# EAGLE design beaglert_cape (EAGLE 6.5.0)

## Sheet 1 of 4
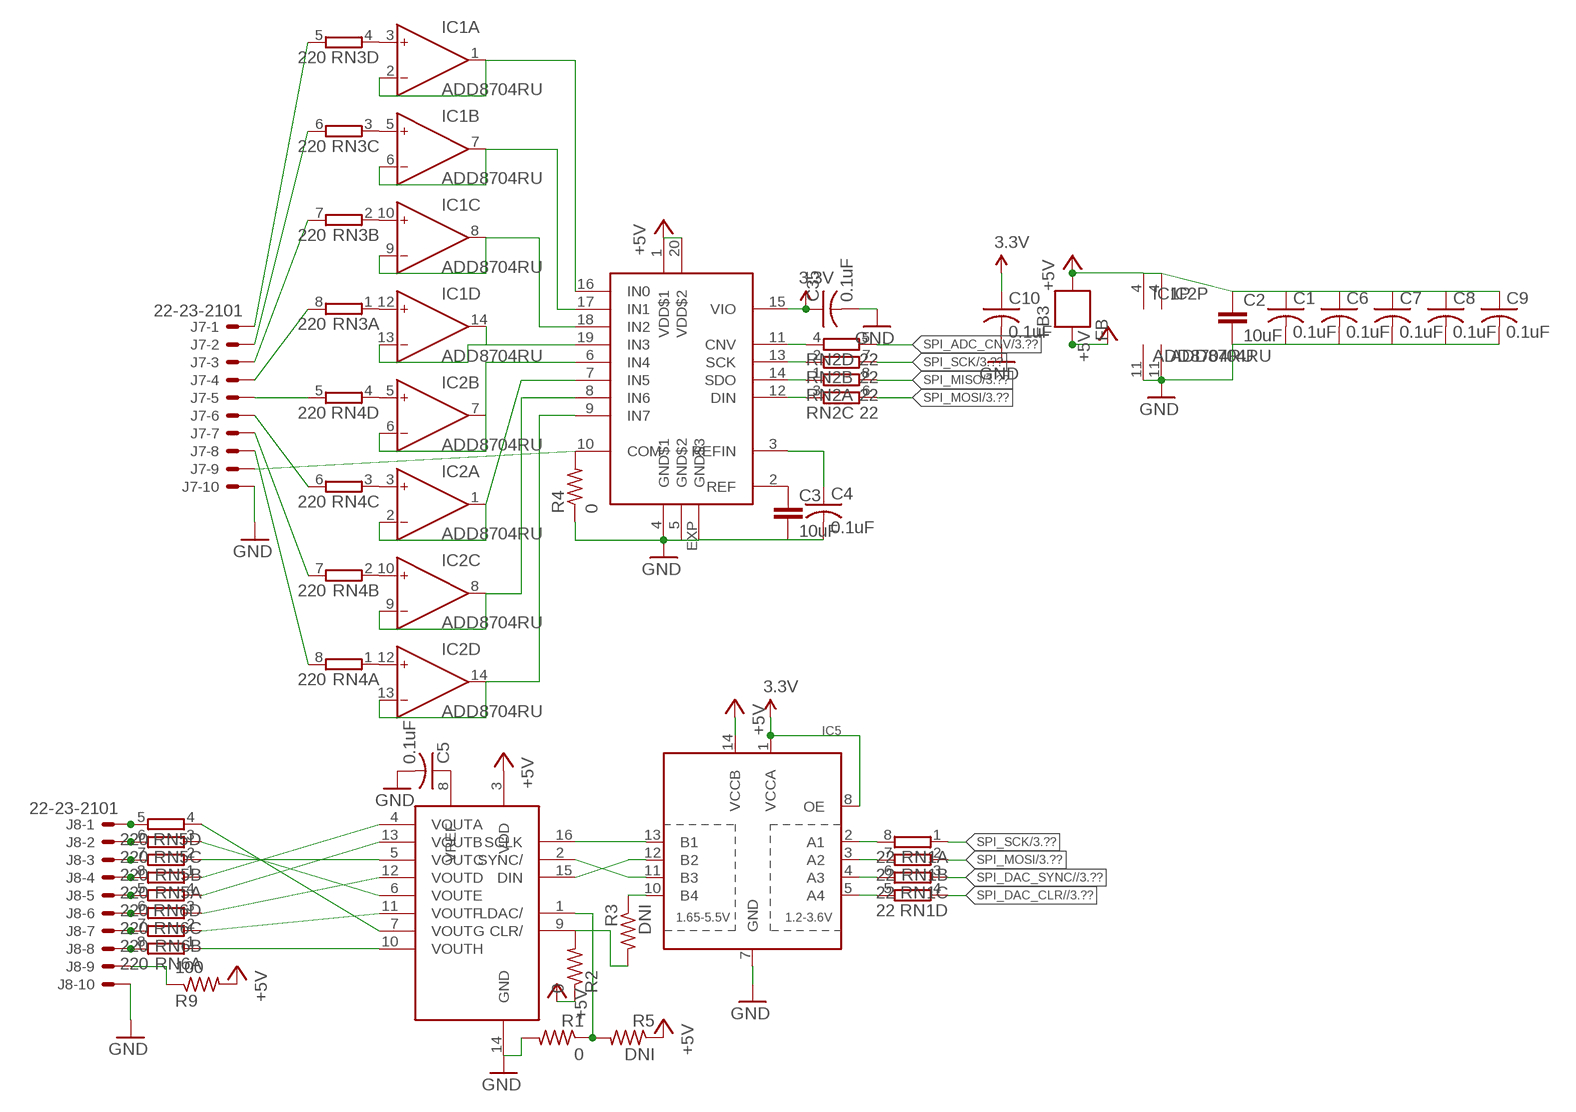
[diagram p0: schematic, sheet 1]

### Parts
C1  0.1uF  C-USC0603  [C0603]
C2  10uF  CAP0603-CAP  [0603-CAP]
C3  10uF  CAP0603-CAP  [0603-CAP]
C4  0.1uF  C-USC0603  [C0603]
C5  0.1uF  C-USC0603  [C0603]
C6  0.1uF  C-USC0603  [C0603]
C7  0.1uF  C-USC0603  [C0603]
C8  0.1uF  C-USC0603  [C0603]
C9  0.1uF  C-USC0603  [C0603]
C10  0.1uF  C-USC0603  [C0603]
C35  0.1uF  C-USC0603  [C0603]
FB3  FB  [0603]
IC1  ADD8704RU  [TSSOP14]
IC2  ADD8704RU  [TSSOP14]
IC3  AD5668  [TSSOP16-PW]
IC4  AD7699  [LFCSP20-LEADS]
IC5  TXB0104PWR  [TSSOP14]
J7  22-23-2101  [22-23-2101]
J8  22-23-2101  [22-23-2101]
R1  0  R-US_R0603  [R0603]
R2  0  R-US_R0603  [R0603]
R3  DNI  R-US_R0603  [R0603]
R4  0  R-US_R0603  [R0603]
R5  DNI  R-US_R0603  [R0603]
R9  100  R-US_R0603  [R0603]
RN1  22  4R-N0603-ARC  [0603-ARC]
RN2  22  4R-N0603-ARC  [0603-ARC]
RN3  220  4R-N0603-ARC  [0603-ARC]
RN4  220  4R-N0603-ARC  [0603-ARC]
RN5  220  4R-N0603-ARC  [0603-ARC]
RN6  220  4R-N0603-ARC  [0603-ARC]

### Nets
3.3V: C10.1 C35.1 IC4.15(VIO) IC5.1(VCCA) IC5.8(OE) ; also sheet 3,4
+5V_ADC_DAC: C1.1 C2.1 C6.1 C7.1 C8.1 C9.1 FB3.1 IC1.4(P:V+) IC2.4(P:V+) IC3.3(VDD) IC4.1(VDD$1) IC4.20(VDD$2) IC5.14(VCCB) R2.1 R5.1 R9.2 ; supply symbol labelled +5V
+5V_SYS: FB3.2 ; supply symbol labelled +5V ; also sheet 3
DGND: C1.2 C2.2 C3.2 C4.2 C5.2 C6.2 C7.2 C8.2 C9.2 C10.2 C35.2 IC1.11(P:V-) IC2.11(P:V-) IC3.14(GND) IC4.4(GND$1) IC4.5(GND$2) IC4.EXP(GND$3) IC5.7(GND) J7.10 J8.10 R1.2 R4.1 ; supply symbol labelled GND ; also sheet 3,4
N$1: IC3.16(SCLK) IC5.13(B1)
N$2: IC3.15(DIN) IC5.12(B2)
N$3: IC3.2(SYNC/) IC5.11(B3)
N$4: IC3.9(CLR/) R2.2 R3.2
N$5: IC1.1(A:OUT) IC1.2(A:IN-) IC4.16(IN0)
N$6: IC1.6(B:IN-) IC1.7(B:OUT) IC4.17(IN1)
N$7: IC1.8(C:OUT) IC1.9(C:IN-) IC4.18(IN2)
N$8: IC1.13(D:IN-) IC1.14(D:OUT) IC4.19(IN3)
N$9: IC2.1(A:OUT) IC2.2(A:IN-) IC4.7(IN5)
N$10: IC2.6(B:IN-) IC2.7(B:OUT) IC4.6(IN4)
N$11: IC2.8(C:OUT) IC2.9(C:IN-) IC4.8(IN6)
N$12: IC2.13(D:IN-) IC2.14(D:OUT) IC4.9(IN7)
N$13: IC5.10(B4) R3.1
N$14: IC4.11(CNV) RN2.4
N$15: C5.1 IC3.8(VREF)
N$16: IC5.2(A1) RN1.8
N$17: IC5.3(A2) RN1.7
N$18: IC5.4(A3) RN1.6
N$19: IC5.5(A4) RN1.5
N$20: IC4.12(DIN) RN2.3
N$21: C3.1 IC4.2(REF)
N$22: C4.1 IC4.3(REFIN)
N$23: IC4.13(SCK) RN2.2
N$24: IC4.14(SDO) RN2.1
N$25: IC4.10(COM) J7.9 R4.2
N$27: IC1.3(A:IN+) RN3.4
N$29: IC1.5(B:IN+) RN3.3
N$30: IC1.10(C:IN+) RN3.2
N$31: IC1.12(D:IN+) RN3.1
N$32: IC2.5(B:IN+) RN4.4
N$33: IC2.3(A:IN+) RN4.3
N$34: IC2.10(C:IN+) RN4.2
N$35: IC2.12(D:IN+) RN4.1
N$36: IC3.1(LDAC/) R1.1 R5.2
N$37: J7.1 RN3.5
N$38: J7.2 RN3.6
N$39: J7.3 RN3.7
N$40: J7.4 RN3.8
N$41: J7.5 RN4.5
N$42: J7.6 RN4.6
N$43: J7.7 RN4.7
N$44: J7.8 RN4.8
N$45: IC3.7(VOUTG) RN5.4
N$46: IC3.6(VOUTE) RN5.3
N$47: IC3.5(VOUTC) RN5.2
N$48: IC3.4(VOUTA) RN5.1
N$49: IC3.13(VOUTB) RN6.4
N$50: IC3.12(VOUTD) RN6.3
N$51: IC3.11(VOUTF) RN6.2
N$52: J8.8 RN6.8
N$61: J8.9 R9.1
N$72: IC3.10(VOUTH) RN6.1
N$73: J8.7 RN6.7
N$74: J8.6 RN6.6
N$75: J8.5 RN6.5
N$76: J8.4 RN5.8
N$77: J8.3 RN5.7
N$78: J8.2 RN5.6
N$79: J8.1 RN5.5
SPI_ADC_CNV: RN2.5 ; also sheet 3
SPI_DAC_CLR/: RN1.4 ; also sheet 3
SPI_DAC_SYNC/: RN1.3 ; also sheet 3
SPI_MISO: RN2.8 ; also sheet 3
SPI_MOSI: RN1.2 RN2.6 ; also sheet 3
SPI_SCK: RN1.1 RN2.7 ; also sheet 3

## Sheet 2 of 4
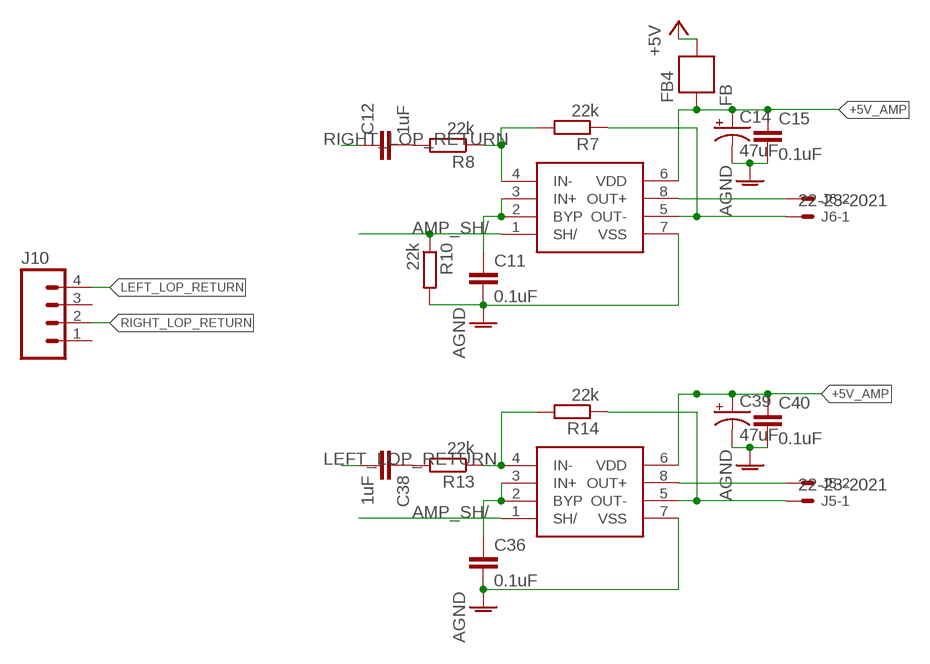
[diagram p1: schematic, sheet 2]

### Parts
C11  0.1uF  C-EUC0603  [C0603]
C12  1uF  C-EUC0603  [C0603]
C14  47uF  CAP_POL1206  [EIA3216]
C15  0.1uF  C-EUC0603  [C0603]
C36  0.1uF  C-EUC0603  [C0603]
C38  1uF  C-EUC0603  [C0603]
C39  47uF  CAP_POL1206  [EIA3216]
C40  0.1uF  C-EUC0603  [C0603]
FB4  FB  [0603]
IC8  LM4876  [SO8]
IC9  LM4876  [SO8]
J5  22-23-2021  [22-23-2021]
J6  22-23-2021  [22-23-2021]
J10  M04PTH  [1X04]
R7  22k  R-EU_R0603  [R0603]
R8  22k  R-EU_R0603  [R0603]
R10  22k  R-EU_R0603  [R0603]
R13  22k  R-EU_R0603  [R0603]
R14  22k  R-EU_R0603  [R0603]

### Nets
+5V_AMP: C14.A(+) C15.1 C39.A(+) C40.1 FB4.2 IC8.6(VDD) IC9.6(VDD)
+5V_POW: FB4.1 ; supply symbol labelled +5V ; also sheet 3
AGND: C11.2 C14.C(-) C15.2 C36.2 C39.C(-) C40.2 IC8.7(VSS) IC9.7(VSS) R10.2 ; also sheet 3
AMP_SH/: IC8.1(SH/) IC9.1(SH/) R10.1 ; also sheet 3
LEFT_LOP_RETURN: C38.2 J10.4
N$26: IC9.4(IN-) R13.1 R14.2
N$28: IC8.4(IN-) R7.2 R8.1
N$53: C11.1 IC8.2(BYP) IC8.3(IN+)
N$55: C12.2 R8.2
N$57: IC8.5(OUT-) J6.1 R7.1
N$60: C36.1 IC9.2(BYP) IC9.3(IN+)
N$64: C38.1 R13.2
N$65: IC9.5(OUT-) J5.1 R14.1
N$67: IC9.8(OUT+) J5.2
N$71: IC8.8(OUT+) J6.2
RIGHT_LOP_RETURN: C12.1 J10.2
Unconnected: J10.1 J10.3

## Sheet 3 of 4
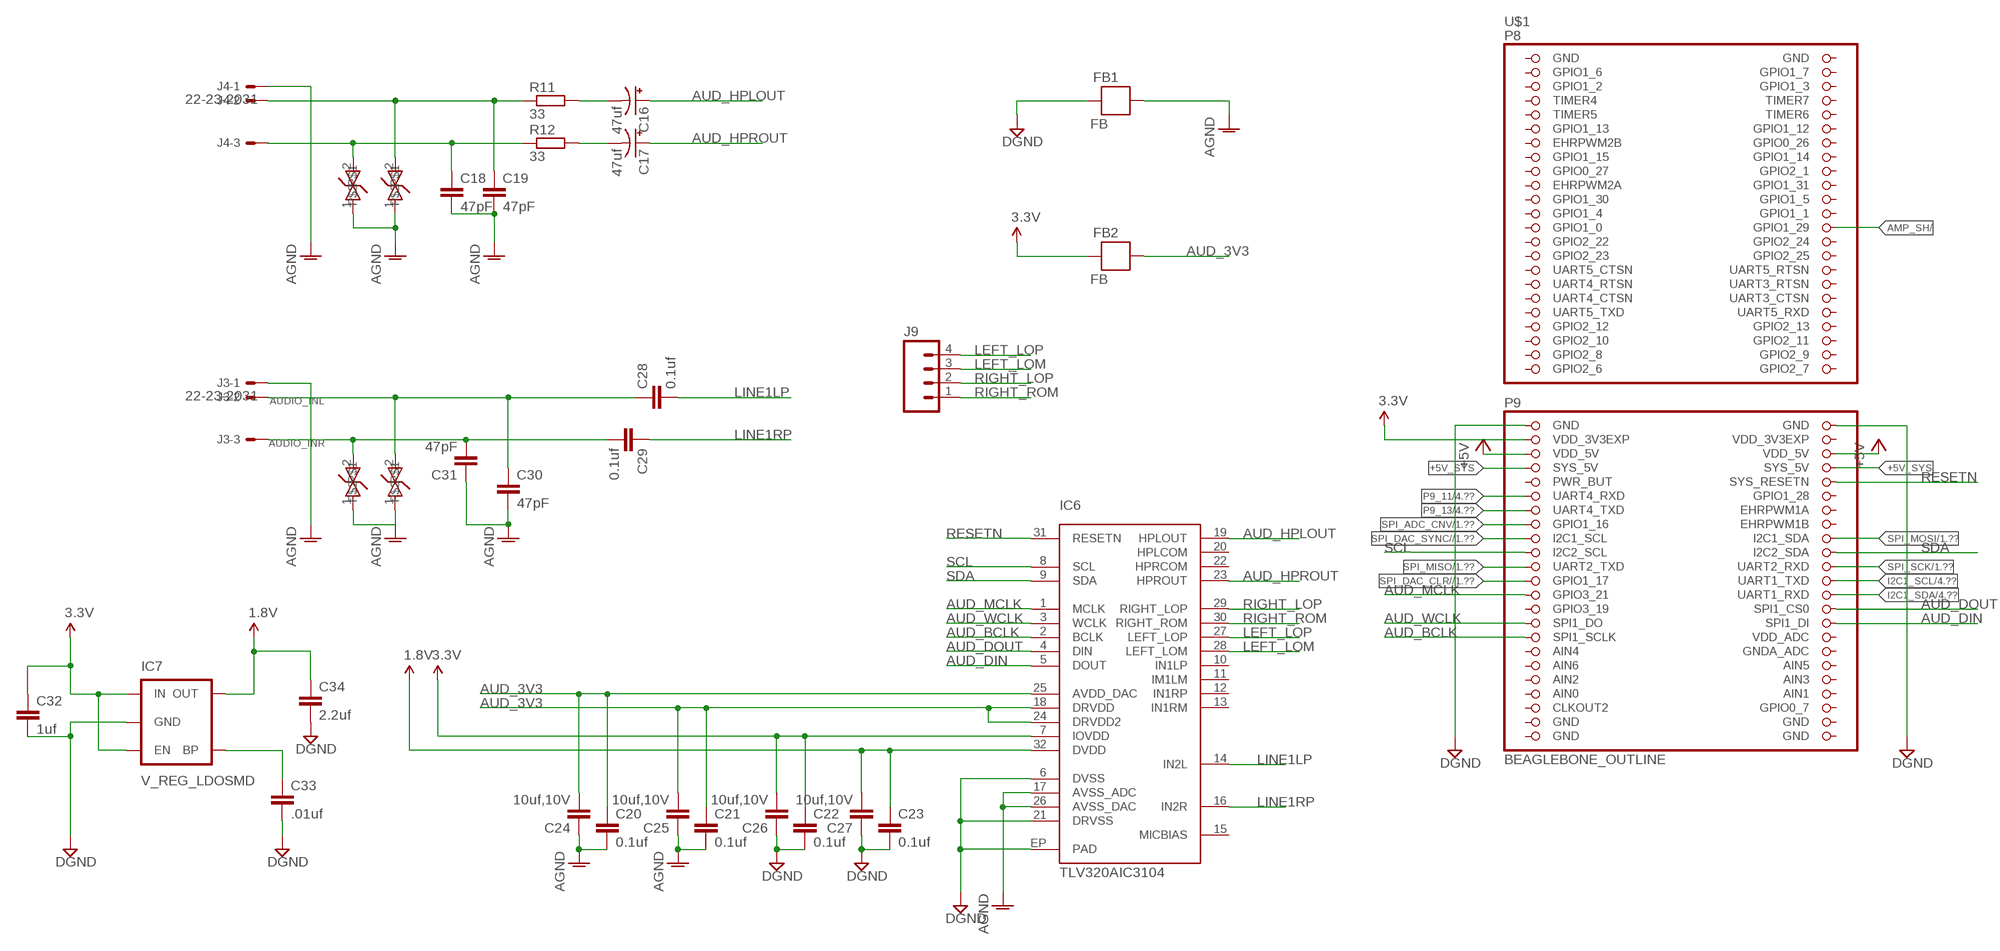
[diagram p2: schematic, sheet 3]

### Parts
C16  47uf  CAP_POL1206  [EIA3216]
C17  47uf  CAP_POL1206  [EIA3216]
C18  47pF  C-EUC0603  [C0603]
C19  47pF  C-EUC0603  [C0603]
C20  0.1uf  C-EUC0603  [C0603]
C21  0.1uf  C-EUC0603  [C0603]
C22  0.1uf  C-EUC0603  [C0603]
C23  0.1uf  C-EUC0603  [C0603]
C24  10uf,10V  CAP0603-CAP  [0603-CAP]
C25  10uf,10V  CAP0603-CAP  [0603-CAP]
C26  10uf,10V  CAP0603-CAP  [0603-CAP]
C27  10uf,10V  CAP0603-CAP  [0603-CAP]
C28  0.1uf  C-EUC0603  [C0603]
C29  0.1uf  C-EUC0603  [C0603]
C30  47pF  C-EUC0603  [C0603]
C31  47pF  C-EUC0603  [C0603]
C32  1uf  C-EUC0603  [C0603]
C33  .01uf  C-EUC0603  [C0603]
C34  2.2uf  C-EUC0603  [C0603]
D1  PGB0010603MR  [0603]
D2  PGB0010603MR  [0603]
D3  PGB0010603MR  [0603]
D4  PGB0010603MR  [0603]
FB1  FB  [0603]
FB2  FB  [0603]
IC6  TLV320AIC3104  [QFN-32]
IC7  V_REG_LDOSMD  [SOT23-5]
J3  22-23-2031  [22-23-2031]
J4  22-23-2031  [22-23-2031]
J9  M04PTH  [1X04]
R11  33  R-EU_R0603  [R0603]
R12  33  R-EU_R0603  [R0603]
U$1  BEAGLEBONE_OUTLINE  [BEAGLEBONE_SHIELD]

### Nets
1.8V: C23.1 C27.2 C34.1 IC6.32(DVDD) IC7.5(OUT)
3.3V: C22.1 C26.2 C32.1 FB2.2 IC6.7(IOVDD) IC7.1(IN) IC7.3(EN) U$1.49(VDD_3V3EXP) ; also sheet 1,4
+5V_POW: U$1.51(VDD_5V) U$1.52(VDD_5V) ; supply symbol labelled +5V ; also sheet 2
+5V_SYS: U$1.53(SYS_5V) U$1.54(SYS_5V) ; also sheet 1
AGND: C18.2 C19.2 C20.2 C21.2 C24.1 C25.1 C30.2 C31.1 D1.1 D2.1 D3.1 D4.1 FB1.1 IC6.17(AVSS_ADC) IC6.26(AVSS_DAC) J3.1 J4.1 ; also sheet 2
AMP_SH/: U$1.26(GPIO1_29) ; also sheet 2
AUD_3V3: C20.1 C21.1 C24.2 C25.2 FB2.1 IC6.18(DRVDD) IC6.24(DRVDD2) IC6.25(AVDD_DAC)
AUD_BCLK: IC6.2(BCLK) U$1.77(SPI1_SCLK)
AUD_DIN: IC6.5(DOUT) U$1.76(SPI1_DI)
AUD_DOUT: IC6.4(DIN) U$1.74(SPI1_CS0)
AUD_HPLOUT: C16.A(+) IC6.19(HPLOUT)
AUD_HPROUT: C17.A(+) IC6.23(HPROUT)
AUD_MCLK: IC6.1(MCLK) U$1.71(GPIO3_21)
AUD_WCLK: IC6.3(WCLK) U$1.75(SPI1_DO)
AUDIO_INL: C28.1 C30.1 D4.2 J3.2
AUDIO_INR: C29.2 C31.2 D3.2 J3.3
DGND: C22.2 C23.2 C26.1 C27.1 C32.2 C33.2 C34.2 FB1.2 IC6.6(DVSS) IC6.21(DRVSS) IC6.EP(PAD) IC7.2(GND) U$1.47(GND) U$1.48(GND) ; also sheet 1,4
HPL: C19.1 D2.2 J4.2 R11.1
HPR: C18.1 D1.2 J4.3 R12.1
I2C1_SCL: U$1.70(UART1_TXD) ; also sheet 4
I2C1_SDA: U$1.72(UART1_RXD) ; also sheet 4
LEFT_LOM: IC6.28(LEFT_LOM) J9.3
LEFT_LOP: IC6.27(LEFT_LOP) J9.4
LINE1LP: C28.2 IC6.14(IN2L)
LINE1RP: C29.1 IC6.16(IN2R)
N$54: C16.C(-) R11.2
N$59: C17.C(-) R12.2
N$63: C33.1 IC7.4(BP)
P9_11: U$1.57(UART4_RXD) ; also sheet 4
P9_13: U$1.59(UART4_TXD) ; also sheet 4
RESETN: IC6.31(RESETN) U$1.56(SYS_RESETN)
RIGHT_LOP: IC6.29(RIGHT_LOP) J9.2
RIGHT_ROM: IC6.30(RIGHT_ROM) J9.1
SCL: IC6.8(SCL) U$1.65(I2C2_SCL)
SDA: IC6.9(SDA) U$1.66(I2C2_SDA)
SPI_ADC_CNV: U$1.61(GPIO1_16) ; also sheet 1
SPI_DAC_CLR/: U$1.69(GPIO1_17) ; also sheet 1
SPI_DAC_SYNC/: U$1.63(I2C1_SCL) ; also sheet 1
SPI_MISO: U$1.67(UART2_TXD) ; also sheet 1
SPI_MOSI: U$1.64(I2C1_SDA) ; also sheet 1
SPI_SCK: U$1.68(UART2_RXD) ; also sheet 1
Unconnected: IC6.10(IN1LP) IC6.11(IM1LM) IC6.12(IN1RP) IC6.13(IN1RM) IC6.15(MICBIAS) IC6.20(HPLCOM) IC6.22(HPRCOM) U$1.3(GPIO1_6) U$1.4(GPIO1_7) U$1.5(GPIO1_2) U$1.6(GPIO1_3) U$1.7(TIMER4) U$1.8(TIMER7) U$1.9(TIMER5) U$1.10(TIMER6) U$1.11(GPIO1_13) U$1.12(GPIO1_12) U$1.13(EHRPWM2B) U$1.14(GPIO0_26) U$1.15(GPIO1_15) U$1.16(GPIO1_14) U$1.17(GPIO0_27) U$1.18(GPIO2_1) U$1.19(EHRPWM2A) U$1.20(GPIO1_31) U$1.21(GPIO1_30) U$1.22(GPIO1_5) U$1.23(GPIO1_4) U$1.24(GPIO1_1) U$1.25(GPIO1_0) U$1.27(GPIO2_22) U$1.28(GPIO2_24) U$1.29(GPIO2_23) U$1.30(GPIO2_25) U$1.31(UART5_CTSN) U$1.32(UART5_RTSN) U$1.33(UART4_RTSN) U$1.34(UART3_RTSN) U$1.35(UART4_CTSN) U$1.36(UART3_CTSN) U$1.37(UART5_TXD) U$1.38(UART5_RXD) U$1.39(GPIO2_12) U$1.40(GPIO2_13) U$1.41(GPIO2_10) U$1.42(GPIO2_11) U$1.43(GPIO2_8) U$1.44(GPIO2_9) U$1.45(GPIO2_6) U$1.46(GPIO2_7) U$1.55(PWR_BUT) U$1.58(GPIO1_28) U$1.60(EHRPWM1A) U$1.62(EHRPWM1B) U$1.73(GPIO3_19) U$1.78(VDD_ADC) U$1.79(AIN4) U$1.80(GNDA_ADC) U$1.81(AIN6) U$1.82(AIN5) U$1.83(AIN2) U$1.84(AIN3) U$1.86(AIN1) U$1.87(CLKOUT2) U$1.88(GPIO0_7)

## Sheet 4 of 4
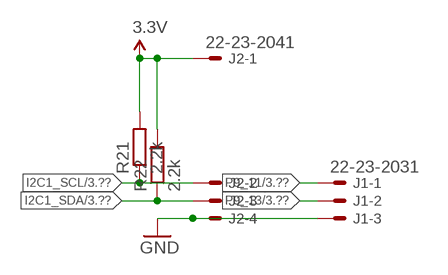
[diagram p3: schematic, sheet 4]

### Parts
J1  22-23-2031  [22-23-2031]
J2  22-23-2041  [22-23-2041]
R21  2.2k  R-EU_R0603  [R0603]
R22  2.2k  R-EU_R0603  [R0603]

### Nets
3.3V: J2.1 R21.2 R22.2 ; also sheet 1,3
DGND: J1.3 J2.4 ; supply symbol labelled GND ; also sheet 1,3
I2C1_SCL: J2.2 R21.1 ; also sheet 3
I2C1_SDA: J2.3 R22.1 ; also sheet 3
P9_11: J1.1 ; also sheet 3
P9_13: J1.2 ; also sheet 3

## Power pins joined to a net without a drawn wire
AIN0: U$1.85(AIN0)
DGND: U$1.1(GND) U$1.2(GND) U$1.89(GND) U$1.90(GND) U$1.91(GND) U$1.92(GND)
VDD_3V3EXP: U$1.50(VDD_3V3EXP)

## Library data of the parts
C1 C4-C10 C35 = rcl:C-US: CAPACITOR, American symbol
C2 C3 = SparkFun-Passives:CAP: Capacitor
C11 C12 C15 C36 C38 C40 = rcl:C-EU: CAPACITOR, European symbol
C14 C39 = SparkFun-Capacitors:CAP_POL: Capacitor Polarized
C16 C17 = SparkFun-Capacitors:CAP_POL: Capacitor Polarized; MANEX: 123-0001196
C18 C19 C30 C31 = rcl:C-EU: CAPACITOR, European symbol; MANEX: 123-0001115
C20-C23 = rcl:C-EU: CAPACITOR, European symbol; MANEX: 123-0001056
C24-C27 = SparkFun-Passives:CAP: Capacitor; MANEX: 123-0001127
C28 C29 C33 = rcl:C-EU: CAPACITOR, European symbol; MANEX: 123-0001032
C32 = rcl:C-EU: CAPACITOR, European symbol; MANEX: 123-0001087
C34 = rcl:C-EU: CAPACITOR, European symbol; MANEX: 123-0001094
D1-D4 = CircuitCo:PGB0010603MR; MANEX: 130-0001371
FB1 FB2 = SparkFun-Passives:FB; MANEX: 126-0001418
FB3 FB4 = SparkFun-Passives:FB
IC1 IC2 = analog-devices:ADD8704: 16 V Quad Operational Amplifier Source: Ananlog Devices .. 780914713ADD8704_0.pdf; MF: ALTERA CORPORATION; MPN: ADD8704ARUZ-REEL; OC_FARNELL: unknown; OC_NEWARK: 59K0964
IC3 = custom:AD5668
IC4 = custom:AD7699
IC5 = SparkFun-DigitalIC:TXB0104PWR: 4-Bit Bi-Directional Level Shifter 1.2V-3.6V (VCCA) to 1.65V-5.5V (VCCB) bi-directional level shifter with auto direction sensing. Max data rate - VCCA 1.8V: 20Mbps (50ns), VCCA 3.3V: 100Mbps (10ns) Digikey: 296-21929-1-ND (TSSOP) IC-11329
IC6 = CircuitCo:TLV320AIC3104; MANEX: 140-0004277
IC7 = SparkFun-PowerIC:V_REG_LDO: Voltage Regulator LDO Standard 150mA LDO voltage regulator in SOT-23 layout. Micrel part MIC5205. BP (by-pass) pin is used to lower output noise with 470pF cap.; MANEX: 140-0001616
IC8 IC9 = custom:LM4876
J1 J3 J4 = con-molex:22-23-2031: .100" (2.54mm) Center Header - 3 Pin; MF: MOLEX; MPN: 22-23-2031; OC_FARNELL: 1462950; OC_NEWARK: 30C0862
J2 = con-molex:22-23-2041: .100" (2.54mm) Center Header - 4 Pin; MF: MOLEX; MPN: 22-23-2041; OC_FARNELL: 1462920; OC_NEWARK: 38C0355
J5 J6 = con-molex:22-23-2021: .100" (2.54mm) Center Header - 2 Pin; MF: MOLEX; MPN: 22-23-2021; OC_FARNELL: 1462926; OC_NEWARK: 25C3832
J7 J8 = con-molex:22-23-2101: .100" (2.54mm) Center Header - 10 Pin; MF: MOLEX; MPN: 22-23-2101; OC_FARNELL: 1756828; OC_NEWARK: 94C0765
J9 J10 = SparkFun-Connectors:M04: Header 4 Standard 4-pin 0.1" header. Use with straight break away headers (SKU : PRT-00116), right angle break away headers (PRT-00553), swiss pins (PRT-00743), machine pins (PRT-00117), and female headers (PRT-00115). Molex polarized connector foot print use with SKU : PRT-08231 with associated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; MANEX: 258-0002845
R1-R5 R9 = rcl:R-US_: RESISTOR, American symbol
R7 R8 R10 R13 R14 R21 R22 = rcl:R-EU_: RESISTOR, European symbol
R11 R12 = rcl:R-EU_: RESISTOR, European symbol; MANEX: 110-0002014
RN1-RN6 = resistor-dil:4R-N: Array Chip Resistor Source: RS Component / Phycomp; OC_FARNELL: unknown; OC_NEWARK: unknown
U$1 = adafruit:BEAGLEBONE_OUTLINE: Should match A3 pinout - but not completely tested

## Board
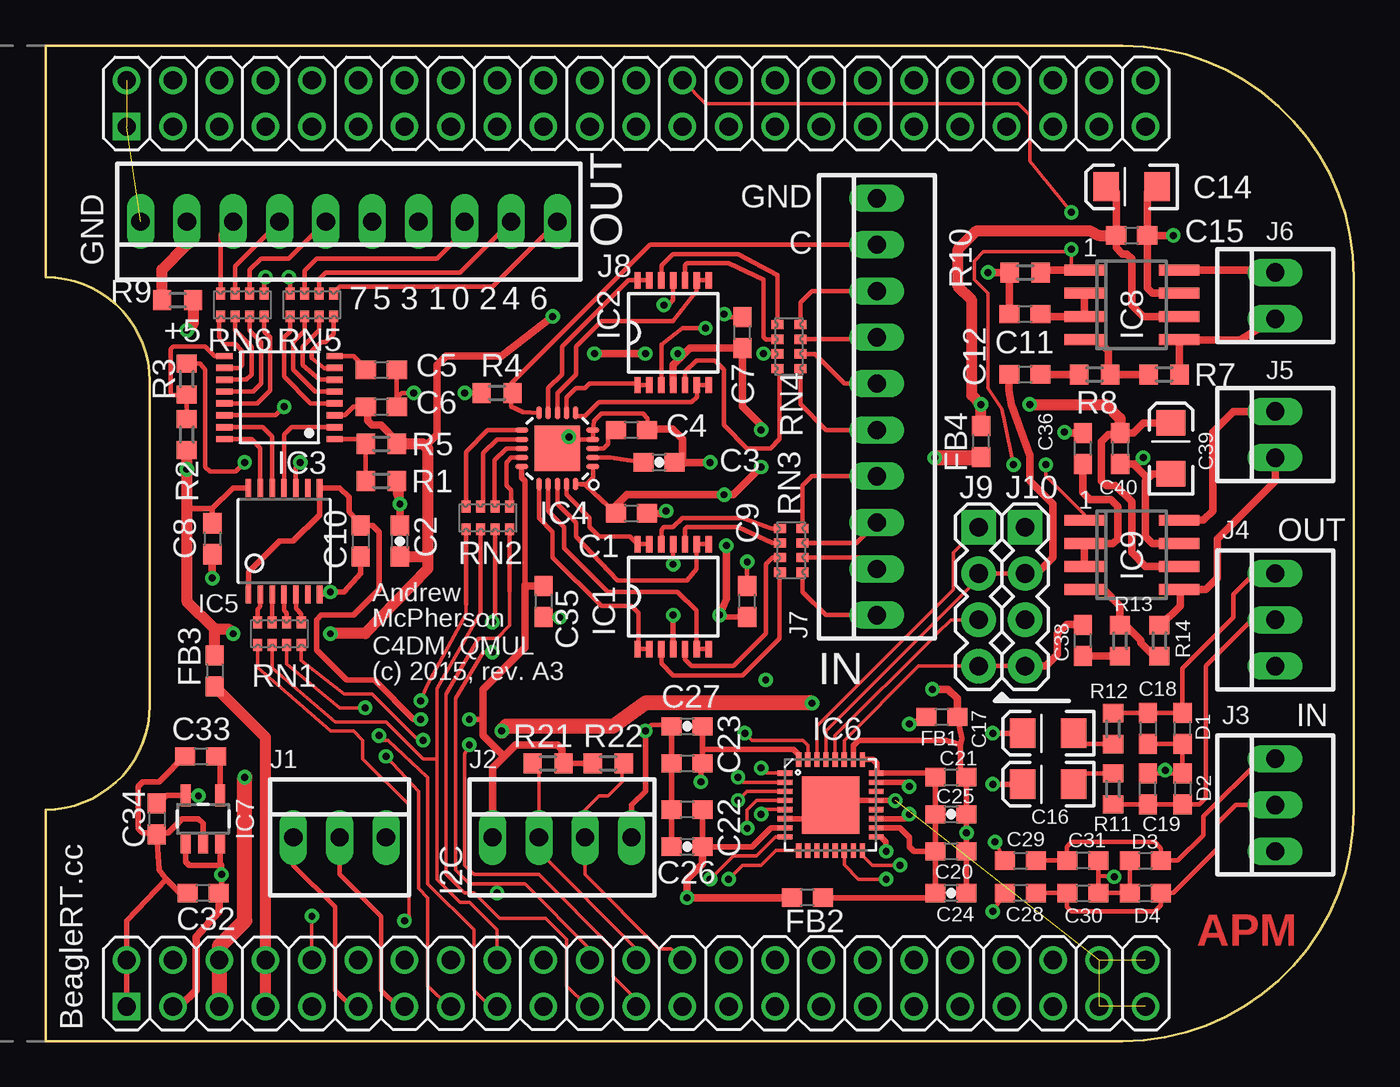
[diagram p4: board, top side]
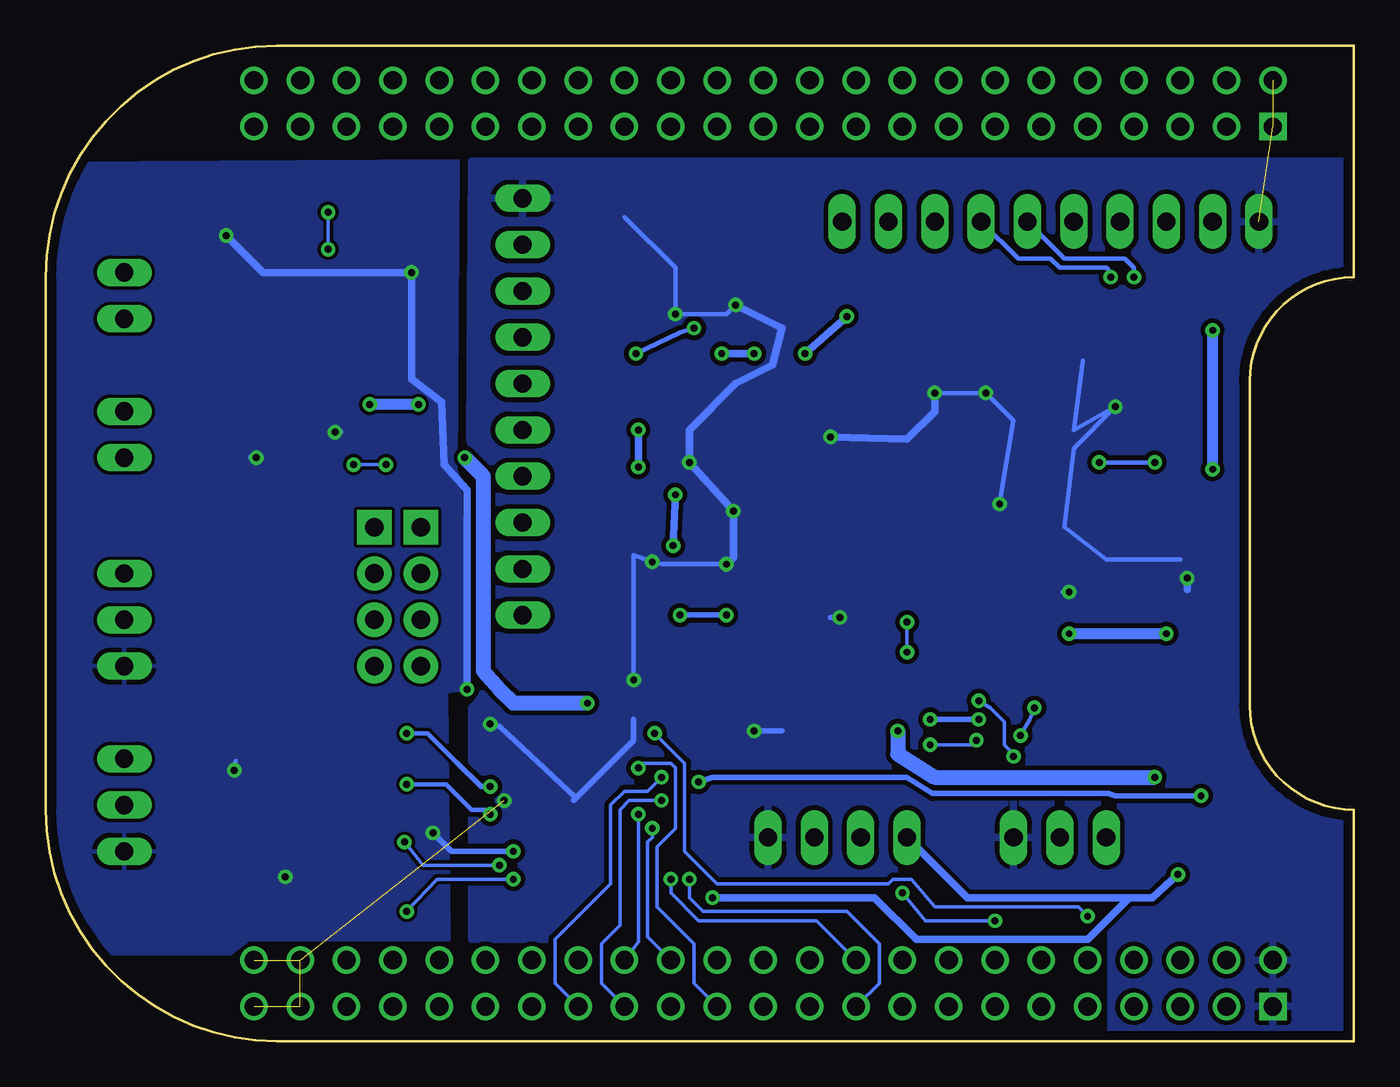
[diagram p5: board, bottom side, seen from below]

Size 71.75 x 54.61 mm. Coordinates in mm from the lower left corner, seen from the top.
Copper layers (1*16): Top 0.035mm / dielectric 1.5mm / Bottom 0.035mm
Design rules "default *": minimum track width 8mil, minimum drill 15mil, track to track 7mil, track to pad 7mil, pad to pad 7mil, via to via 7mil, smd to smd 0mil, copper to edge 20mil, drill to drill 8mil, minimum pad ring 10mil, minimum via ring 8mil, stop-mask expansion 4mil, vias tented up to drill 0mil, thermal gap 10mil

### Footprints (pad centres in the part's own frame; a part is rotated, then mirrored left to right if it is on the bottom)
C0603 = smd 1.1 x 1: 1 -0.85,0; 2 0.85,0
0603-CAP = smd 1.1 x 1: 1 -0.85,0; 2 0.85,0
EIA3216 = smd 1.4 x 1.6: A 1.4,0; C -1.4,0
0603 = smd 1.1 x 1: 1 -0.85,0; 2 0.85,0
TSSOP14 = smd 0.9 x 0.35: 1 -2.875,1.95; 2 -2.875,1.3; 3 -2.875,0.65; 4 -2.875,0; 5 -2.875,-0.65; 6 -2.875,-1.3; 7 -2.875,-1.95; 8 2.875,-1.95; 9 2.875,-1.3; 10 2.875,-0.65; 11 2.875,0; 12 2.875,0.65; 13 2.875,1.3; 14 2.875,1.95
TSSOP16-PW = smd 0.35 x 0.9: 1 -2.275,-3.025; 2 -1.625,-3.025; 3 -0.975,-3.025; 4 -0.325,-3.025; 5 0.325,-3.025; 6 0.975,-3.025; 7 1.625,-3.025; 8 2.275,-3.025; 9 2.275,3.025; 10 1.625,3.025; 11 0.975,3.025; 12 0.325,3.025; 13 -0.325,3.025; 14 -0.975,3.025; 15 -1.625,3.025; 16 -2.275,3.025
LFCSP20-LEADS = smd 0.7 x 0.3: 1 -1.95,1; 2 -1.95,0.5; 3 -1.95,0; 4 -1.95,-0.5; 5 -1.95,-1; 11 1.95,-1; 12 1.95,-0.5; 13 1.95,0; 14 1.95,0.5; 15 1.95,1 | smd 0.3 x 0.7: 6 -1,-1.95; 7 -0.5,-1.95; 8 0,-1.95; 9 0.5,-1.95; 10 1,-1.95; 16 1,1.95; 17 0.5,1.95; 18 0,1.95; 19 -0.5,1.95; 20 -1,1.95 | smd 2.5 x 2.5: EXP 0,0
TSSOP14' = smd 0.305 x 0.991: 1 -1.95,-2.918; 2 -1.3,-2.918; 3 -0.65,-2.918; 4 0,-2.918; 5 0.65,-2.918; 6 1.3,-2.918; 7 1.95,-2.918; 8 1.95,2.918; 9 1.3,2.918; 10 0.65,2.918; 11 0,2.918; 12 -0.65,2.918; 13 -1.3,2.918; 14 -1.95,2.918
QFN-32 = smd 0.285 x 0.8: 1 -1.75,-2.5; 2 -1.25,-2.5; 3 -0.75,-2.5; 4 -0.25,-2.5; 5 0.25,-2.5; 6 0.75,-2.5; 7 1.25,-2.5; 8 1.75,-2.5; 17 1.75,2.5; 18 1.25,2.5; 19 0.75,2.5; 20 0.25,2.5; 21 -0.25,2.5; 22 -0.75,2.5; 23 -1.25,2.5; 24 -1.75,2.5 | smd 0.8 x 0.285: 9 2.5,-1.75; 10 2.5,-1.25; 11 2.5,-0.75; 12 2.5,-0.25; 13 2.5,0.25; 14 2.5,0.75; 15 2.5,1.25; 16 2.5,1.75; 25 -2.5,1.75; 26 -2.5,1.25; 27 -2.5,0.75; 28 -2.5,0.25; 29 -2.5,-0.25; 30 -2.5,-0.75; 31 -2.5,-1.25; 32 -2.5,-1.75 | smd 3.15 x 3.15: EP 0,0
SOT23-5 = smd 0.55 x 1.2: 1 -0.95,-1.3; 2 0,-1.3; 3 0.95,-1.3; 4 0.95,1.3; 5 -0.95,1.3
SO8 = smd 0.6 x 2.2: 1 -1.905,-2.6; 2 -0.635,-2.6; 3 0.635,-2.6; 4 1.905,-2.6; 5 1.905,2.6; 6 0.635,2.6; 7 -0.635,2.6; 8 -1.905,2.6
22-23-2031 = drill 1 long: 1 -2.54,0; 2 0,0; 3 2.54,0
22-23-2041 = drill 1 long: 1 -3.81,0; 2 -1.27,0; 3 1.27,0; 4 3.81,0
22-23-2021 = drill 1 long: 1 -1.27,0; 2 1.27,0
22-23-2101 = drill 1 long: 1 -11.43,0; 2 -8.89,0; 3 -6.35,0; 4 -3.81,0; 5 -1.27,0; 6 1.27,0; 7 3.81,0; 8 6.35,0; 9 8.89,0; 10 11.43,0
1X04 = drill 1.016 pad 1.88 square: 1 0,0 | drill 1.016 pad 1.88: 2 2.54,0; 3 5.08,0; 4 7.62,0
R0603 = smd 1 x 1.1: 1 -0.85,0; 2 0.85,0
0603-ARC = smd 0.5 x 0.65: 1 -1.2,-0.625; 2 -0.4,-0.625; 3 0.4,-0.625; 4 1.2,-0.625; 5 1.2,0.625; 6 0.4,0.625; 7 -0.4,0.625; 8 -1.2,0.625
BEAGLEBONE_SHIELD = drill 1 square: 1 4.445,19.05; 47 52.705,19.05 | drill 1: 2 1.905,19.05; 3 4.445,21.59; 4 1.905,21.59; 5 4.445,24.13; 6 1.905,24.13; 7 4.445,26.67; 8 1.905,26.67; 9 4.445,29.21; 10 1.905,29.21; 11 4.445,31.75; 12 1.905,31.75; 13 4.445,34.29; 14 1.905,34.29; 15 4.445,36.83; 16 1.905,36.83; 17 4.445,39.37; 18 1.905,39.37; 19 4.445,41.91; 20 1.905,41.91; 21 4.445,44.45; 22 1.905,44.45; 23 4.445,46.99; 24 1.905,46.99; 25 4.445,49.53; 26 1.905,49.53; 27 4.445,52.07; 28 1.905,52.07; 29 4.445,54.61; 30 1.905,54.61; 31 4.445,57.15; 32 1.905,57.15; 33 4.445,59.69; 34 1.905,59.69; 35 4.445,62.23; 36 1.905,62.23; 37 4.445,64.77; 38 1.905,64.77; 39 4.445,67.31; 40 1.905,67.31; 41 4.445,69.85; 42 1.905,69.85; 43 4.445,72.39; 44 1.905,72.39; 45 4.445,74.93; 46 1.905,74.93; 48 50.165,19.05; 49 52.705,21.59; 50 50.165,21.59; 51 52.705,24.13; 52 50.165,24.13; 53 52.705,26.67; 54 50.165,26.67; 55 52.705,29.21; 56 50.165,29.21; 57 52.705,31.75; 58 50.165,31.75; 59 52.705,34.29; 60 50.165,34.29; 61 52.705,36.83; 62 50.165,36.83; 63 52.705,39.37; 64 50.165,39.37; 65 52.705,41.91; 66 50.165,41.91; 67 52.705,44.45; 68 50.165,44.45; 69 52.705,46.99; 70 50.165,46.99; 71 52.705,49.53; 72 50.165,49.53; 73 52.705,52.07; 74 50.165,52.07; 75 52.705,54.61; 76 50.165,54.61; 77 52.705,57.15; 78 50.165,57.15; 79 52.705,59.69; 80 50.165,59.69; 81 52.705,62.23; 82 50.165,62.23; 83 52.705,64.77; 84 50.165,64.77; 85 52.705,67.31; 86 50.165,67.31; 87 52.705,69.85; 88 50.165,69.85; 89 52.705,72.39; 90 50.165,72.39; 91 52.705,74.93; 92 50.165,74.93

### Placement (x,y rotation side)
C1  32.13,28.96 0 top
C2  19.43,27.43 90 top
C3  33.66,31.75 0 top
C4  32.13,33.53 0 top
C5  18.41,36.83 0 top
C6  18.41,34.8 0 top
C7  38.23,38.86 90 top
C8  9.14,27.56 270 top
C9  38.48,24.13 90 top
C10  17.27,27.43 270 top
C11  53.72,39.88 180 top
C12  53.72,36.58 0 top
C14  59.56,46.86 180 top
C15  59.56,44.2 0 top
C16  54.99,14.1 180 top
C17  54.99,16.89 180 top
C18  60.45,17.15 270 top
C19  60.45,13.84 90 top
C20  49.66,10.41 0 top
C21  49.66,14.48 0 top
C22  35.18,12.7 180 top
C23  35.18,15.24 180 top
C24  49.66,8.13 180 top
C25  49.66,12.45 180 top
C26  35.18,10.67 0 top
C27  35.18,17.27 0 top
C28  53.47,8.13 180 top
C29  53.47,9.91 0 top
C30  56.9,8.13 0 top
C31  56.9,9.91 180 top
C32  8.64,8.13 180 top
C33  8.51,15.62 180 top
C34  6.1,12.19 270 top
C35  27.3,24.13 270 top
C36  56.9,32.51 90 top
C38  56.9,21.97 90 top
C39  61.72,32.51 90 top
C40  58.93,32.51 270 top
D1  62.36,17.15 90 top
D2  62.36,13.84 270 top
D3  60.33,9.91 0 top
D4  60.33,8.13 0 top
FB1  49.15,17.78 180 top
FB2  41.78,7.87 180 top
FB3  9.27,20.32 270 top
FB4  51.31,32.89 90 top
IC1  34.42,24.38 90 top
IC2  34.42,38.86 90 top
IC3  12.83,35.31 90 top
IC4  28.07,32.51 180 top
IC5  [TSSOP14']  13.08,27.43 0 top
IC6  43.05,12.95 270 top
IC7  8.64,12.19 0 top
IC8  59.56,40.39 270 top
IC9  59.56,26.67 270 top
J1  16.13,11.18 0 top
J2  28.32,11.18 0 top
J3  67.44,12.95 90 top
J4  67.44,23.11 90 top
J5  67.44,33.27 90 top
J6  67.44,40.89 90 top
J7  45.59,34.8 90 top
J8  16.64,44.96 180 top
J9  51.18,28.19 270 top
J10  53.72,28.19 270 top
R1  18.41,30.73 0 top
R2  7.75,33.27 90 top
R3  7.75,36.32 270 top
R4  24.77,35.56 0 top
R5  18.41,32.77 180 top
R7  61.34,36.58 180 top
R8  57.53,36.58 180 top
R9  7.24,40.64 0 top
R10  53.72,42.16 180 top
R11  58.55,13.84 90 top
R12  58.55,17.15 270 top
R13  58.93,21.97 270 top
R14  61.09,21.97 270 top
R21  27.56,15.24 0 top
R22  30.86,15.24 180 top
RN1  12.83,22.35 0 top
RN2  24.26,28.7 180 top
RN3  40.89,26.92 270 top
RN4  40.77,38.1 270 top
RN5  14.61,40.39 0 top
RN6  10.8,40.39 0 top
U$1  -14.61,54.61 270 top

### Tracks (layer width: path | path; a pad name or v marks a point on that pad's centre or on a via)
1.8V  (via drill 0.38)
  Top 0.305: C27.2 36.03,16 | 36.03,16 C23.1 35.94,15.15 v35.94,14.22 | IC6.32 41.3,15.72 41.02,16 36.03,16 | C34.1 6.67,13.49 IC7.5 7.84,13.49 v8.38,13.46
  Bottom 0.305: v8.38,13.46 13.08,13.46 13.46,13.59 23.11,13.59 24.51,14.48 35.18,14.48 v35.94,14.22
3.3V  (via drill 0.38)
  Top 0.305: IC6.7 39.77,11.7 38.73,10.67 C26.2 C22.1 | IC7.1 7.69,9.84 7.87,9.65 9.65,9.65 | 9.65,9.65 v9.65,9.14 9.65,8.29 C32.1 9.53,8.09 9.53,8.04 | IC7.3 9.59,9.72 9.65,9.65 | R22.2 R21.2 28.32,15.33 | IC5.1 11.13,25.74 12.83,27.43 13.59,27.43 15.03,28.87 IC5.8 16.13,30.35 16.64,29.84 16.64,29.04 C10.1 17.95,28.28 18.29,27.94 18.29,24.77 16.89,23.37 15.11,23.37 14.86,23.11 14.86,21.46 16.51,19.81 18.03,19.81 20.19,17.65 v20.57,17.65 | IC4.15 26.12,30.91 26.29,30.73 26.29,25.02 26.33,24.98 | v23.24,17.65 23.88,17.65 24,17.78
  Top 0.406: U$1.49 7.37,1.91 8.26,2.79 8.26,5.72 9.53,7.11 9.53,8.04 | FB2.2 v35.18,7.87 35.18,8.89 36.03,9.74 C26.2 | 9.49,7.87 C32.1 | J2.1 24.51,14.99 25.15,15.62 | 25.15,15.62 25.78,16.26 28.07,16.26 28.32,16 28.32,15.33 | 26.29,25.02 26.29,21.59 24,19.3 24,17.78 24,16.76 25.15,15.62 | C35.1 26.33,24.98
  Bottom 0.305: v20.57,17.65 v23.24,17.65
  Bottom 0.406: v35.18,7.87 26.29,7.87 24,5.59 14.61,5.59 12.32,7.87 | J2.1 21.21,7.87 12.32,7.87 | 12.32,7.87 11.05,7.87 v9.65,9.14
+5V_ADC_DAC  (via drill 0.38, 0.38 pad 0.41)
  Top 0.254: C1.1 29.6,30.51 IC4.20 29.67,30.56 30.02,30.91 IC4.1 | 8.09,32.42 R2.1 | IC3.3 16.42,34.33 16.89,34.8 C6.1 17.65,34.71 | R5.1 19.27,32.93
  Top 0.305: C9.1 37.05,23.28 v36.96,23.37 | v34.42,23.37 IC1.4 | IC5.14 10.28,30.35 9.14,29.21 | 9.14,29.21 C8.1 | 9.14,29.21 7.87,29.21 7.75,29.34
  Top 0.406: 19.27,32.93 18.41,33.78 17.91,33.78 17.65,34.04 17.65,34.71 | 34.8,37.47 35.34,38.01 C7.1 38.23,34.8 39.24,33.78 v39.24,33.53 | 34.8,37.47 34.42,37.08 IC2.4 | C1.1 31.28,29.38 31.88,29.97 v37.21,29.97 37.72,29.97 v39.24,31.5 | C9.1 38.57,23.37 | 20.96,32.51 20.96,32.77 21.46,33.27 21.46,37.08 21.97,37.59 25.02,37.59 v27.81,39.75 | v32.89,37.72 v30.1,37.72 | v36.96,23.37 37.34,24.26 v37.34,27.18 | 34.8,37.47 v34.67,37.72
  Top 0.61: v15.62,22.35 17.53,22.35 20.96,25.91 20.96,26.42 | R5.1 20.7,32.77 20.96,32.51 20.96,26.42 | R2.1 7.71,32.42 v7.75,31.37 7.75,29.34 7.75,24.13 9.27,22.61 | R9.2 8.09,39.33 v7.75,38.99 | C2.1 20.87,26.58 20.96,26.42 | FB3.1 9.27,22.61 | 9.27,22.61 10.03,22.61 v10.29,22.35
  Bottom 0.305: v36.96,23.37 v34.42,23.37
  Bottom 0.406: v39.24,33.53 v39.24,31.5 | v37.21,29.97 v37.34,27.18 | v34.67,37.72 v32.89,37.72 | v30.1,37.72 v27.81,39.75
  Bottom 0.61: v15.62,22.35 v10.29,22.35 | v7.75,31.37 v7.75,38.99
+5V_AMP  (via drill 0.38)
  Top 0.406: C15.1 58.71,43.52 59.05,43.18 59.31,43.18 59.56,42.93 59.56,40.39 60.2,39.75 IC8.6 | C15.1 58.71,46.57 58.55,46.74 C14.A | 58.46,44.45 C15.1 | IC9.6 60.33,26.04 59.56,26.8 59.56,29.59 58.67,30.48 58.17,30.48 57.91,30.73 57.91,32.89 58.29,33.27 58.84,33.27 C40.1 59.65,33.36 60.2,33.91 C39.A
  Top 0.61: C15.1 57.79,44.2 57.28,44.45 51.05,44.45 50.04,43.43 50.04,41.4 50.8,40.64 50.8,35.43 v51.31,34.92 FB4.2 | v53.98,34.92 58.17,34.92 58.93,34.16 C40.1
  Bottom 0.61: v51.31,34.92 v53.98,34.92
+5V_POW  (via drill 0.38)
  Top 0.813: U$1.51 U$1.52 9.53,5.21 10.92,6.6 v10.92,14.48 | v42.04,18.54 32.89,18.54 31.12,17.27 25.27,17.27 v25.02,17.02 | v48.77,32 51.27,32 FB4.1
  Bottom 0.254: 46.86,19.3 46.86,19.05
  Bottom 0.813: v10.92,14.48 22.99,14.48 25.02,15.75 v25.02,17.02 | v42.04,18.54 46.1,18.54 46.86,19.3 47.75,20.32 47.75,30.99 v48.77,32
+5V_SYS
  Top 0.61: U$1.53 U$1.54 12.07,16.68 FB3.2
AGND  (via drill 0.38)
  Top 0.254: 57.75,9.06 C30.2 D4.1 D3.1 | C31.1 57.75,9.06 | 57.75,9.06 v58.61,9.02 | C18.2 D1.1 D2.1 C19.2 61.18,14.69 v61.4,14.86
  Top 0.305: IC6.26 44.3,16.24 44.58,16.51 49.4,16.51 50.16,16.26 | 50.16,16.26 50.16,14.57 C21.2 C25.1 C20.2 v50.51,11.43 C24.1 | IC6.17 45.82,11.2 46.1,10.92 v46.1,10.41 | FB1.1 50.25,16.6 50.16,16.26
  Top 0.406: FB1.1 50,18.8 49.49,19.3 v48.64,19.3 | C11.2 R10.2 v51.69,42.16 | C15.2 60.41,41.31 60.71,41.02 IC8.7 | C15.2 60.41,46.57 60.83,46.74 C14.C | v61.85,44.2 C15.2 | IC9.7 60.71,27.3 60.33,27.69 60.33,30.73 60.45,30.86 | C39.C 60.7,31.11 60.45,30.86 | 60.45,30.86 59.65,31.66 C40.2 59.86,31.66 v60.2,32 | C36.2 55.92,33.36 v55.88,33.4
  Bottom 0.254: v58.61,9.02 58.55,9.02 | v61.4,14.86 61.34,15.37
  Bottom 0.305: v46.1,10.41 49.49,10.41 v50.51,11.43
  Bottom 0.406: v61.85,44.2 59.82,42.16 v51.69,42.16 51.69,36.32 50.04,35.05 49.91,31.62 48.64,30.23 v48.64,19.3 | v55.88,33.4 55.63,33.4 | v60.2,32 60.45,32
  pour Bottom: 49.66,5.59 60.58,5.59 61.59,4.83 71.5,4.83 70.99,48.13 49.15,48.26 49.28,31.24 49.02,30.73 48.77,19.3 49.78,19.18
AMP_SH/  (via drill 0.38)
  Top 0.203: v56.26,45.47 53.98,48.26 53.98,50.8 53.34,51.44 36.2,51.44 U$1.26 | 56.26,42.29 v56.26,43.43 56.13,43.31 51.44,43.31 50.93,42.8 50.93,41.78 51.69,41.02 51.69,35.81 52.45,34.67 v53.09,31.62 | IC9.1 56.96,28.89 54.86,30.99 v54.86,31.62
  Top 0.406: IC8.1 56.26,42.29 54.7,42.29 R10.1
  Bottom 0.203: v56.26,45.47 v56.26,43.43 | v54.86,31.62 v53.09,31.62
AUD_3V3
  Top 0.305: FB2.1 48.3,7.87 C24.2 C20.1 | C20.1 C25.2 C21.1 48.33,14.7 IC6.24 45.59,14.74 45.59,15.24 45.38,15.45 IC6.25 | IC6.18 46.84,11.7 47.37,11.18 47.37,10.67 47.62,10.41 C20.1
AUD_BCLK  (via drill 0.38)
  Top 0.203: IC6.2 38.25,14.2 v37.97,14.48
  Bottom 0.203: v37.97,14.48 38.73,13.72 40.01,13.72 40.77,12.95 40.77,8.64 43.81,5.59 43.81,3.17 U$1.77
AUD_DIN  (via drill 0.38)
  Top 0.203: IC6.5 39.5,12.7 v39.24,12.45
  Bottom 0.203: v39.24,12.45 39.24,5.46 U$1.76
AUD_DOUT  (via drill 0.38)
  Top 0.203: IC6.4 38.98,13.2 38.48,12.7 v38.48,11.68
  Bottom 0.203: v38.48,11.68 38.48,11.18 38.73,10.92 38.73,5.72 U$1.74
AUD_HPLOUT  (via drill 0.38)
  Top 0.203: 53.08,13.59 C16.A
  Top 0.305: IC6.19 47.13,12.2 v47.37,12.45 | v51.94,14.1 C16.A
  Bottom 0.254: 47.37,12.7 48.39,12.7 49.78,14.1 v51.94,14.1
  Bottom 0.305: v47.37,12.45 47.37,12.7
AUD_HPROUT  (via drill 0.38)
  Top 0.305: IC6.23 47.14,14.2 v47.37,13.97 | v51.94,16.89 C17.A
  Bottom 0.254: 49.15,15.24 50.8,16.89 v51.94,16.89
  Bottom 0.305: v47.37,13.97 47.88,13.97 49.15,15.24
AUD_MCLK  (via drill 0.38)
  Top 0.203: IC6.1 39.52,14.7 v39.24,14.99
  Bottom 0.203: v39.24,14.99 38.99,15.24 37.47,15.24 37.21,14.99 37.21,11.68 38.23,10.67 38.23,7.37 36.2,5.33 36.2,3.17 U$1.71
AUD_WCLK  (via drill 0.38)
  Top 0.203: IC6.3 38.47,13.7 v37.97,13.21
  Bottom 0.203: v37.97,13.21 39.75,13.21 40.26,12.7 40.26,6.35 41.27,5.33 41.27,3.17 U$1.75
AUDIO_INL
  Top 0.254: C28.1 C30.1 56.01,8.09 56.01,7.37 56.26,7.11 60.83,7.11 61.18,7.45 D4.2 61.85,8.13 64.26,10.54 64.26,11.94 65.28,12.95 J3.2
AUDIO_INR
  Top 0.203: C29.2 54.48,9.91
  Top 0.254: C29.2 C31.2 56.01,9.95 56.01,10.67 56.26,10.92 60.83,10.92 61.18,10.58 D3.2 62.1,9.91 63.5,11.3 63.5,12.32 66.68,15.49 J3.3
DGND  (via drill 0.38, 0.38 pad 0.41)  (6 unrouted)
  Top 0.254: IC4.EXP 28.57,33.01 IC4.4 IC4.5 30.07,34.01 30.48,34.42 32.77,34.42 33.02,34.16 33.02,33.57 C4.2 | 19.27,35.31 C5.2 | 19.27,35.31 C6.2 | R1.2 19.43,30.57 | IC3.14 12.61,34.33 v13.08,34.8 | v22.99,35.56 R4.1 | v20.19,35.56 19.52,35.56 19.27,35.31 | C7.2 37.38,39.71 v37.21,39.88 | v33.91,40.39 34.16,40.39 34.42,40.64 IC2.11 | v38.48,26.29 C9.2 | v34.42,26.16 IC1.11 | 34.42,17.36 33.23,17.36 v32.89,17.02 | IC5.7 15.5,24.51 v15.62,24.64
  Top 0.305: IC6.6 42.3,12.2 IC6.EP 43.3,13.2 IC6.21 v46.61,13.2 | C34.2 6.22,9.4 6.6,8.89 | 6.6,8.89 7.37,8.13 C32.2 | IC7.2 8.64,11.94 8.38,12.19 7.49,12.19 6.73,11.43 6.31,11.43 C34.2 | C33.2 7.75,15.75 6.22,14.22 5.33,14.22 5.08,13.97 5.08,11.68 5.33,11.43 6.14,11.43 C34.2 | 6.6,8.89 4.45,6.6 U$1.48 U$1.47 | C26.1 C22.2 C23.2 C27.1 34.42,17.36 | FB1.2 v47.37,17.4 | J2.4 32.13,12.95 32.89,13.72 v32.89,17.02 | C10.2 17.27,25.65 16.38,24.64 v15.62,24.64 | C35.2 28.16,23.28 v28.19,23.24
  Top 0.406: 19.43,30.57 C2.2 | R1.2 19.27,30.06 v19.43,29.46 | IC4.EXP v28.7,33.15 | 33.02,33.57 34.38,33.57 34.92,33.02 34.92,31.62 C3.2 v36.45,31.75 | C1.2 33.91,28.96 v34.04,29.08 | C8.2 v9.14,25.4
  Bottom 0.254: 14.86,37.34 15.37,33.53 v13.08,34.8 15.37,32.51 15.88,28.19 13.59,26.42 9.53,26.42 | v22.99,35.56 v20.19,35.56 18.67,34.04 v19.43,29.46 | v33.91,40.39 34.42,39.88 v37.21,39.88 37.21,42.42 40.01,45.21 | v39.5,19.81 39.5,26.67 v38.48,26.29 37.97,26.16 v34.42,26.16 | v15.62,24.64 16,24.64
  Bottom 0.305: 42.8,13.21 42.67,13.34 | 42.67,13.34 39.5,16.51 39.5,17.65 | v47.37,17.4 46.86,17.27 42.67,13.34 | v32.89,17.02 31.37,17.02 | v28.19,23.24 28.7,23.24
  Bottom 0.406: v28.7,33.15 24.51,33.02 22.99,34.54 v22.99,35.56 | v34.42,26.16 34.04,26.54 v34.04,29.08 v36.45,31.75 36.45,33.53 33.91,36.07 31.88,37.08 31.37,39.12 v33.91,40.39 | v9.14,25.4 9.14,24.77
  pour Bottom (isolate 0.254): 48.39,48.26 0.38,48.26 0.38,0.51 13.34,0.51 13.34,7.87 41.02,7.87 41.02,5.59 48.39,5.59 48.39,18.29 48.01,18.67 47.88,30.99 48.51,33.02
HPL
  Top 0.254: R11.1 C19.1 D2.2 63.29,12.99 63.63,13.34 63.63,20.57 66.17,23.11 J4.2
HPR
  Top 0.254: R12.1 C18.1 D1.2 62.36,20.45 65.15,23.24 65.15,24.51 66.29,25.65 J4.3
I2C1_SCL
  Top 0.203: U$1.70 32.39,5.08 27.05,10.41 J2.2 27.05,14.9 R21.1
I2C1_SDA
  Top 0.203: U$1.72 34.29,5.08 33.66,5.08 29.59,9.14 J2.3 29.59,12.7 30.35,13.46 30.86,13.46 31.62,14.22 31.62,15.15 R22.1
LEFT_LOM
  Top 0.203: IC6.28 43.3,16.76 48.64,22.1 48.9,22.35 49.66,23.11 J9.3
LEFT_LOP
  Top 0.203: IC6.27 43.8,16.5 47.88,20.57 J9.4
LEFT_LOP_RETURN
  Top 0.254: J10.4 51.18,20.57
  Top 0.406: C38.2 56.86,22.86 56.01,22.86 55.5,22.35 55.5,21.21 54.86,20.57 J10.4
LINE1LP  (via drill 0.38)
  Top 0.203: IC6.14 43.8,9.66 44.58,8.89 v46.1,8.89 | v51.94,7.11 C28.2
  Bottom 0.203: v46.1,8.89 50.29,8.89 v51.94,7.11
LINE1RP  (via drill 0.38)
  Top 0.203: IC6.16 44.8,10.19 45.34,9.65 v46.86,9.65 | v52.07,10.92 C29.1
  Bottom 0.203: v46.86,9.65 51.05,9.65 v52.07,10.92
N$1
  Top 0.254: IC3.16 11.29,33.03 11.78,32.54 IC5.13
N$2
  Top 0.254: IC3.15 11.91,33.68 12.43,33.16 IC5.12
N$3
  Top 0.254: IC3.2 13.49,33.68 13.08,33.27 IC5.11
N$4
  Top 0.254: R2.2 R3.2 7.71,35.43 6.99,35.43 6.86,35.56 6.86,37.97 6.99,38.1 8.76,38.1 9.28,37.58 IC3.9
N$5
  Top 0.254: IC1.2 IC1.1 32.51,21.55 32.51,23.49 32.13,23.88 30.48,23.88 27.81,26.54 27.81,27.94 27.07,28.69 IC4.16
N$6
  Top 0.254: IC4.17 27.57,29.08 28.45,28.19 28.45,27.05 30.86,24.64 34.67,24.64 35.69,23.62 35.69,21.54 IC1.6 IC1.7
N$7
  Top 0.254: IC4.18 28.07,29.46 29.08,28.45 29.08,27.69 31.37,25.27 35.18,25.27 35.69,25.91 35.69,27.23 IC1.9 IC1.8
N$8
  Top 0.254: IC4.19 28.57,29.98 29.85,28.7 29.85,28.19 30.35,27.69 32.04,27.69 IC1.14 IC1.13
N$9
  Top 0.254: IC2.2 IC2.1 | IC2.1 32.47,36.24 | IC4.7 28.57,35.3 29.08,35.81 29.59,35.81 29.85,36.07 32.39,36.07 IC2.1
N$10
  Top 0.254: IC2.7 IC2.6 35.72,35.34 35.43,35.05 30.35,35.05 29.59,34.29 29.1,34.29 IC4.6
N$11
  Top 0.254: IC4.8 28.07,35.56 29.08,36.58 29.08,38.1 30.48,39.5 34.42,39.5 35.69,41.15 35.69,41.71 IC2.9 IC2.8
N$12
  Top 0.254: IC2.13 IC2.14 31.96,41.74 28.32,38.1 28.32,36.58 27.56,35.81 27.56,34.27 IC4.9
N$13  (via drill 0.38)
  Top 0.254: R3.1 8.47,37.17 8.76,36.83 8.76,31.5 9.02,31.24 10.41,31.24 v10.92,31.75 | v13.97,31.75 13.72,31.5 13.72,30.37 IC5.10
  Bottom 0.254: v10.92,31.75 v13.97,31.75
N$14
  Top 0.254: IC4.11 24.24,33.51 23.06,32.33 RN2.4
N$15
  Top 0.254: C5.1 17.57,36.92 16.89,37.59 15.86,37.59 IC3.8
N$16
  Top 0.254: IC5.2 11.78,23.85 11.63,23.69 RN1.8
N$17
  Top 0.254: 12.5,23.05 RN1.7 IC5.3
N$18
  Top 0.254: 13.15,23.05 RN1.6 13.23,23.48 13.08,23.62 IC5.4
N$19
  Top 0.254: IC5.5 13.73,23.73 14.03,23.44 RN1.5
N$20
  Top 0.254: IC4.12 24.76,33.01 24,32.26 24,29.47 RN2.3
N$21
  Top 0.254: IC4.2 30.98,32.01 C3.1
N$22
  Top 0.254: IC4.3 30.61,32.51 30.86,32.77 30.86,33.11 C4.1
N$23
  Top 0.254: IC4.13 25.27,32.51 24.64,31.88 24.64,29.31 RN2.2
N$24
  Top 0.254: IC4.14 25.54,32.01 25.27,31.75 25.27,30.48 25.53,30.23 25.53,29.4 RN2.1
N$25
  Top 0.254: IC4.10 26.19,34.52 25.53,34.8 25.53,35.47 R4.2 25.53,35.65 25.53,36.07 33.15,43.69 J7.9
N$26
  Top 0.406: R14.2 60.79,21.12 60.07,21.84 60.07,21.97 59.22,22.82 R13.1 58.93,23.88 58.04,24.77 IC9.4
N$27
  Top 0.254: IC1.3 33.77,20.72 34.42,20.07 38.23,20.07 40.26,22.1 RN3.4
N$28
  Top 0.406: IC8.4 57.66,38.48 58.29,37.85 58.29,36.66 | R8.1 R7.2
  Top 0.61: R8.1 58.29,36.66
N$29
  Top 0.254: IC1.5 35.07,20.94 35.43,20.57 37.72,20.57 39.5,22.35 39.5,26.16 39.86,26.52 RN3.3
N$30
  Top 0.254: IC1.10 35.07,28.08 35.18,28.19 37.97,28.19 39.86,27.32 RN3.2
N$31
  Top 0.254: IC1.12 33.77,28.05 33.91,28.19 34.42,28.19 34.92,28.7 38.23,28.7 39.82,28.12 RN3.1
N$32
  Top 0.254: IC2.5 35.07,36.72 35.69,37.34 36.7,37.34 37.21,36.83 37.21,33.78 38.48,32.51 39.75,32.51 40.26,33.02 40.26,36.78 RN4.4
N$33  (via drill 0.38)
  Top 0.254: IC2.3 33.77,38.21 34.92,39.12 v36.2,39.12 | v39.37,37.72 40.12,37.72 RN4.3
  Bottom 0.254: v36.2,39.12 36.96,38.86 v39.37,37.72
N$34
  Top 0.254: IC2.10 35.07,42.56 35.18,42.67 37.47,42.67 39.37,41.78 39.37,38.61 39.5,38.48 40.12,38.48 RN4.2
N$35
  Top 0.254: IC2.12 33.77,42.53 34.42,43.18 37.97,43.18 40.14,42.03 RN4.1
N$36
  Top 0.254: IC3.1 17.3,33.03 R5.2 R1.1
N$37
  Top 0.254: RN3.5 41.52,24.65 42.8,23.37 J7.1
N$38
  Top 0.254: RN3.6 44.98,26.52 J7.2
N$39
  Top 0.254: RN3.7 44.47,27.32 J7.3
N$40
  Top 0.254: RN3.8 41.52,30.47 42.04,30.99 J7.4
N$41
  Top 0.254: RN4.5 41.39,34.94 42.8,33.53 J7.5
N$42
  Top 0.254: RN4.6 42.18,37.7 43.81,36.07 J7.6
N$43
  Top 0.254: RN4.7 45.48,38.5 J7.7
N$44
  Top 0.254: RN4.8 41.39,40.5 42.04,41.15 J7.8
N$45
  Top 0.254: IC3.7 15.27,36.93 14.61,37.47 14.61,37.85 15.11,38.35 15.37,38.35 15.81,38.79 RN5.4
N$46
  Top 0.254: IC3.6 15.03,36.28 14.1,37.08 14.1,38.1 15.01,39.01 RN5.3
N$47
  Top 0.254: IC3.5 14.79,35.63 13.59,36.83 13.59,38.35 14.21,38.97 RN5.2
N$48
  Top 0.254: IC3.4 14.55,34.98 13.08,36.45 13.08,38.61 13.41,38.93 RN5.1
N$49
  Top 0.254: IC3.13 11.61,34.98 12.32,35.69 12.32,38.61 12,38.93 RN6.4
N$50
  Top 0.254: IC3.12 11.37,35.63 11.81,36.07 11.81,38.35 11.2,38.97 RN6.3
N$51
  Top 0.254: IC3.11 11.01,36.28 11.3,36.58 11.3,38.1 10.4,39.01 RN6.2
N$52
  Top 0.254: RN6.8 9.6,44.27 J8.8
N$53
  Top 0.406: C11.1 54.7,39.75 IC8.3 IC8.2
N$54
  Top 0.254: R11.2 56.99,14.69 C16.C
N$55
  Top 0.406: R8.2 C12.2
N$57
  Top 0.406: R7.1 62.19,38.45 | 62.19,38.45 IC8.5 | 62.19,38.45 65.5,38.45 J6.1
N$59
  Top 0.254: R12.2 56.99,16.3 C17.C
N$60
  Top 0.406: IC9.3 IC9.2 58.55,27.3 58.8,27.56 58.8,29.34 58.42,29.72 57.28,29.72 56.9,30.1 C36.1
N$61
  Top 0.61: R9.1 6.39,42.33 7.75,43.69 J8.9
N$63
  Top 0.305: IC7.4 9.59,15.39 C33.1
N$64
  Top 0.406: R13.2 C38.1
N$65
  Top 0.406: R14.1 61.18,22.82 62.23,23.88 62.23,24.7 IC9.5 63.63,24.77 64.26,25.4 64.26,27.56 67.44,30.73 J5.1
N$67
  Top 0.406: IC9.8 63.5,28.58 64.01,29.08 64.01,33.4 65.15,34.54 J5.2
N$71
  Top 0.406: IC8.8 66.55,42.29 J6.2
N$72
  Top 0.254: IC3.10 10.64,36.93 10.8,37.08 10.8,37.85 10.41,38.23 9.78,38.23 9.53,38.61 9.53,39.69 RN6.1
N$73
  Top 0.254: RN6.7 10.4,42.53 J8.7
N$74
  Top 0.254: RN6.6 11.2,42.31 11.81,42.93 13.34,42.93 J8.6
N$75  (via drill 0.38)
  Top 0.254: RN6.5 12,41.84 v12.07,41.91
  Bottom 0.254: v12.07,41.91 12.07,42.42 12.57,42.93 15.88,42.93 J8.5
N$76  (via drill 0.38)
  Top 0.254: RN5.8 13.41,41.84 v13.34,41.91
  Bottom 0.254: v13.34,41.91 13.34,42.16 13.59,42.42 16.13,42.42 16.64,42.93 18.41,42.93 J8.4
N$77
  Top 0.254: RN5.7 14.21,42.27 14.86,42.93 21.46,42.93 22.99,44.45 J8.3
N$78
  Top 0.254: RN5.6 15.01,41.8 15.37,42.16 22.73,42.16 J8.2
N$79
  Top 0.254: RN5.5 15.81,41.08 16.13,41.4 24.51,41.4 J8.1
P9_11
  Top 0.254: U$1.57 16.76,1.91 15.88,2.79 15.88,7.37 13.59,9.65 J1.1
P9_13
  Top 0.254: U$1.59 19.3,1.91 18.41,2.79 18.41,6.86 16.13,9.14 J1.2
RESETN  (via drill 0.38)
  Top 0.203: U$1.56 v14.61,6.86 | IC6.31 41.8,16.24 41.53,16.51 38.73,16.51 v38.35,16.89
  Bottom 0.203: v14.61,6.86 15.11,7.37 22.99,7.37 24.26,8.89 25.27,8.89 25.53,8.64 34.92,8.64 36.7,10.41 36.7,15.24 v38.35,16.89
RIGHT_LOP
  Top 0.203: IC6.29 42.8,17.02 51.18,25.4 J9.2
RIGHT_LOP_RETURN
  Top 0.254: J10.2 51.18,25.65
  Top 0.406: C12.1 52.83,36.54 52.83,35.69 52.96,34.92 53.98,32.13 53.98,30.73 55.25,29.46 55.25,26.54 54.36,25.65 J10.2
RIGHT_ROM
  Top 0.203: IC6.30 42.3,17.28 49.78,24.77 49.78,26.8 J9.1
SCL  (via drill 0.38)
  Top 0.203: IC6.8 40.03,11.2 38.99,10.16 37.72,10.16 v36.45,8.89
  Bottom 0.203: v36.45,8.89 36.45,7.87 35.69,7.11 27.81,7.11 26.04,5.33 26.04,3.17 U$1.65
SDA  (via drill 0.38)
  Top 0.203: IC6.9 40.05,10.45 39.24,9.65 38.23,9.65 v37.47,8.89
  Bottom 0.203: v37.47,8.89 37.47,8.13 35.94,6.6 29.46,6.6 U$1.66
SPI_ADC_CNV  (via drill 0.38)
  Top 0.203: U$1.61 22.1,1.91 20.96,3.05 20.96,7.87 20.45,8.38 20.45,13.72 v18.67,15.62 | 23.06,23.95 23.06,23.44 20.96,19.56 v20.57,18.67
  Top 0.254: RN2.5 23.06,23.95
  Bottom 0.203: v20.57,18.67 19.94,18.29 19.18,17.53 19.18,16.26 18.67,15.75 v18.67,15.62
SPI_DAC_CLR/  (via drill 0.38)
  Top 0.203: U$1.69 32.39,2.29 31.12,3.56 31.12,5.08 27.05,9.14 23.5,9.14 22.99,9.65 22.99,15.75 v23.24,16.26 | v20.7,16.51 20.45,16.51 17.91,19.05 16.38,19.05 14.03,20.9 RN1.4
  Bottom 0.203: v23.24,16.26 20.96,16.26 v20.7,16.51
SPI_DAC_SYNC/  (via drill 0.38)
  Top 0.203: U$1.63 24.38,1.91 23.5,2.79 23.5,6.1 20.96,8.64 20.96,14.48 18.8,16.51 18.54,16.51 v18.29,16.76 | RN1.3 13.23,20.68 16.13,18.29 v17.53,18.29
  Bottom 0.203: v18.29,16.76 17.78,17.65 v17.53,18.29
SPI_MISO
  Top 0.203: U$1.67 29.72,1.91 28.58,3.05 28.58,5.59 27.43,6.73 24.89,6.73 23.5,8.13 22.99,8.13 21.97,9.14 21.97,19.05 23.75,22.1 24.77,22.1 25.46,22.79 25.46,24.71
  Top 0.254: RN2.8 25.46,24.71
SPI_MOSI
  Top 0.203: U$1.64 24.77,6.1 23.24,7.62 22.73,7.62 21.46,8.89 21.46,15.49 | 21.46,15.49 21.46,19.34 23.86,23.51 | RN1.2 12.43,20.47 15.88,17.53 18.67,17.53 20.7,15.49 21.46,15.49
  Top 0.254: RN2.6 23.86,23.51
SPI_SCK  (via drill 0.38)
  Top 0.203: U$1.68 29.85,5.08 26.29,8.64 24.77,8.64 | 24.77,8.64 23.24,8.64 22.48,9.4 22.48,18.8 24,21.34 v24.51,21.34 | RN1.1 11.63,20.5 15.62,17.02 16.89,17.02 17.4,16.51 17.4,15.49 19.94,12.95 19.94,6.86 v19.69,6.6 | v24.77,8.13 24.77,8.64
  Top 0.254: RN2.7 24.66,23.26 v24.51,22.99
  Bottom 0.203: v24.51,22.99 v24.51,21.34 | v19.69,6.6 23.5,6.6 v24.77,8.13

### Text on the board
Top: APM
tPlace: OUT | GND | GND | C | 1 | 7 | 5 | 3 | 1 | 0 | 2 | 4 | 6 | +5 | 1 | OUT | Andrew | McPherson | C4DM, QMUL | IN | (c) 2015, rev. A3 | IN | I2C | BeagleRT.cc

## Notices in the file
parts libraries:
SparkFun-Capacitors: Licensing: CC v3.0 Share-Alike You are welcome to use this library for commercial purposes.
